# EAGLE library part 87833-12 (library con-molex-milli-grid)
HEADER
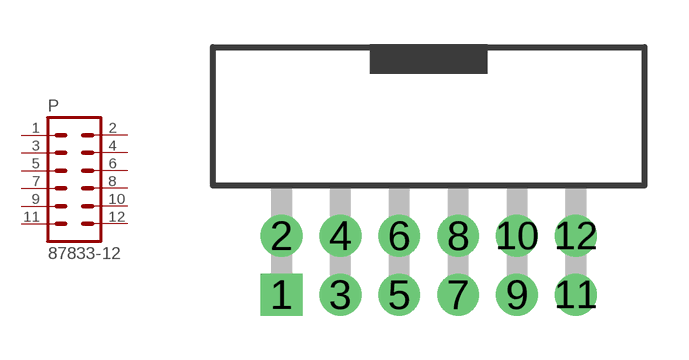
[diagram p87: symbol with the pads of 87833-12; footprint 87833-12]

Designator prefix P

## 87833-12  [87833-12]
1  1  pas
2  2  pas
3  3  pas
4  4  pas
5  5  pas
6  6  pas
7  7  pas
8  8  pas
9  9  pas
10  10  pas
11  11  pas
12  12  pas

## Footprint 87833-12 (pad centres in mm)
HEADER Dual Row, Shrouded, Right Angle
drill 0.914 square: 1 -5,-1
drill 0.914: 2 -5,1; 3 -3,-1; 4 -3,1; 5 -1,-1; 6 -1,1; 7 1,-1; 8 1,1; 9 3,-1; 10 3,1; 11 5,-1; 12 5,1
